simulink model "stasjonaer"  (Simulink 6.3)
settings: Solver=ode23tb  StartTime=0.0  StopTime=simtid  MaxStep=10  RelTol=1e-6  AbsTol=1e-6
InitFcn:
  | Exp_data;
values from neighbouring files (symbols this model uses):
  mG_in = 0.362    [finn_TF.m]    (also in null_pol_forflytning.m; slug_3D_lin.m = u(2); slug_3D_sim.m = u(2); s_slug.m)
  mL_in = 8.64    [finn_TF.m]    (also in null_pol_forflytning.m; slug_3D_lin.m = u(3); slug_3D_sim.m = u(3); s_slug.m)
  z_arbpkt = 70    [finn_TF.m]    (also in null_pol_forflytning.m)
  z_setpkt = 0.175    [finn_TF.m]    (also in null_pol_forflytning.m = z_vec(jj))
libraries: simulink_extras x2

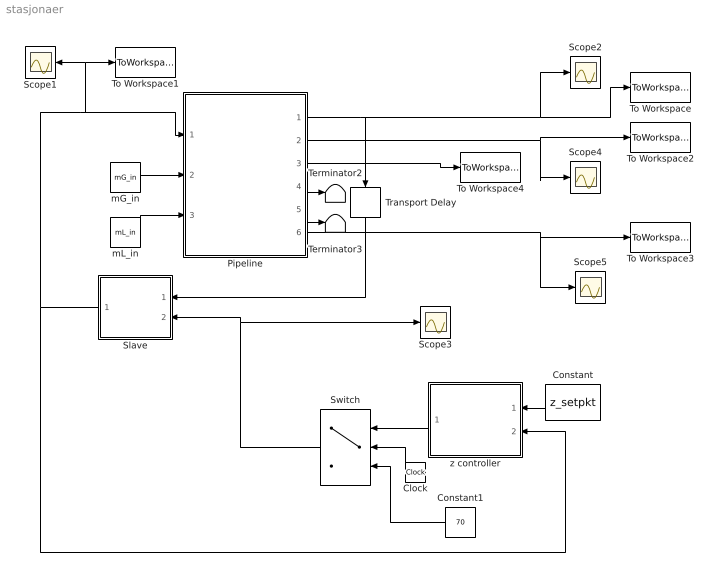
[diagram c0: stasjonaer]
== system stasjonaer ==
  Clock : Clock
  Constant : Constant  Orientation=left  Value=z_setpkt
  Constant1 : Constant  Orientation=left  Value=70
  Pipeline : Subsystem
  Scope{1..5} (5 alike) : Scope
  Slave : Subsystem  Orientation=left
  Switch : Switch  Orientation=left
  Terminator2 : Terminator
  Terminator3 : Terminator
  To Workspace : ToWorkspace  VariableName=P1_simulert  SampleTime=-1  SaveFormat=Structure With Time
  To Workspace1 : ToWorkspace  VariableName=z  SampleTime=-1  SaveFormat=Structure With Time
  To Workspace2 : ToWorkspace  VariableName=P2_simulert  SampleTime=-1  SaveFormat=Structure With Time
  To Workspace3 : ToWorkspace  VariableName=h1_simulert  SampleTime=-1  SaveFormat=Structure With Time
  To Workspace4 : ToWorkspace  VariableName=rhoT_simulert  SampleTime=-1  SaveFormat=Structure With Time
  Transport Delay : TransportDelay  Orientation=down  InitialOutput=1
  mG_in : Constant  Value=mG_in
  mL_in : Constant  Value=mL_in
  z controller : Subsystem  Orientation=left
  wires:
  Pipeline/1(P1) -> Transport Delay/1, To Workspace/1, Scope2/1
  Transport Delay/1 -> Slave/1(measurement)
  Pipeline/2("P2 ") -> To Workspace2/1, Scope4/1
  Pipeline/3("rho_T ") -> To Workspace4/1
  Pipeline/4(W) -> Terminator2/1
  Pipeline/5(Q) -> Terminator3/1
  mL_in/1 -> Pipeline/3(mL_in)
  mG_in/1 -> Pipeline/2(mG_in)
  Slave/1(z) -> Pipeline/1(z), To Workspace1/1, Scope1/1, z controller/2("measurement  z ")
  Constant/1 -> z controller/1("sett.pkt z ")
  Clock/1 -> Switch/2
  z controller/1("ref. pressure cont. ") -> Switch/1
  Constant1/1 -> Switch/3
  Switch/1 -> Slave/2(ref), Scope3/1
  Pipeline/6(h1) -> To Workspace3/1, Scope5/1

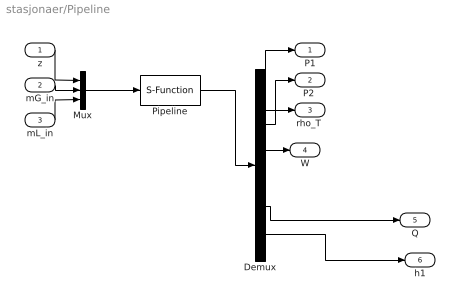
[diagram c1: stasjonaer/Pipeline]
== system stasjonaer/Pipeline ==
  z : Inport
  mG_in : Inport  Port=2
  mL_in : Inport  Port=3
  Demux : Demux  Outputs=6
  Mux : Mux  Inputs=3
  Pipeline : S-Function  FunctionName=s_slug
  P1 : Outport
  "P2 " : Outport  Port=2
  "rho_T " : Outport  Port=3
  W : Outport  Port=4
  Q : Outport  Port=5
  h1 : Outport  Port=6
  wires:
  Pipeline/1 -> Demux/1
  Mux/1 -> Pipeline/1
  Demux/1 -> P1/1
  z/1 -> Mux/1
  mG_in/1 -> Mux/2
  Demux/2 -> "P2 "/1
  mL_in/1 -> Mux/3
  Demux/3 -> "rho_T "/1
  Demux/4 -> W/1
  Demux/5 -> Q/1
  Demux/6 -> h1/1

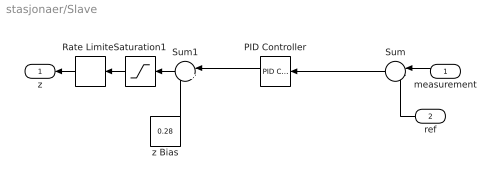
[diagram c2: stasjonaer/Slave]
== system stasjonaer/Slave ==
  measurement : Inport  Orientation=left
  ref : Inport  Orientation=left  Port=2
  PID Controller : simulink_extras/Additional Linear/PID Controller  Orientation=left  P=-0.5  I=-0.5/600  D=0
  Rate Limiter : RateLimiter  Orientation=left  RisingSlewLimit=1/60  FallingSlewLimit=-1/60
  Saturation1 : Saturate  Orientation=left  UpperLimit=1  LowerLimit=0.02
  Sum : Sum  Orientation=left  Inputs=|-+
  Sum1 : Sum  Orientation=left  Inputs=|++
  z Bias : Constant  Value=0.28
  z : Outport  Orientation=left
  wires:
  Sum/1 -> PID Controller/1
  z Bias/1 -> Sum1/2
  measurement/1 -> Sum/1
  ref/1 -> Sum/2
  Rate Limiter/1 -> z/1
  PID Controller/1 -> Sum1/1
  Sum1/1 -> Saturation1/1
  Saturation1/1 -> Rate Limiter/1

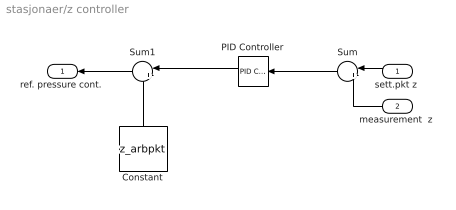
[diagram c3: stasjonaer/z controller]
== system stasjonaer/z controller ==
  "sett.pkt z " : Inport  Orientation=left
  "measurement  z " : Inport  Orientation=left  Port=2
  Constant : Constant  Orientation=up  Value=z_arbpkt
  PID Controller : simulink_extras/Additional Linear/PID Controller  Orientation=left  P=-11.2  I=-11.2/510  D=0
  Sum : Sum  Orientation=left  Inputs=|+-
  Sum1 : Sum  Orientation=left  Inputs=|++
  "ref. pressure cont. " : Outport  Orientation=left
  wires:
  Sum/1 -> PID Controller/1
  "sett.pkt z "/1 -> Sum/1
  "measurement  z "/1 -> Sum/2
  PID Controller/1 -> Sum1/1
  Sum1/1 -> "ref. pressure cont. "/1
  Constant/1 -> Sum1/2
